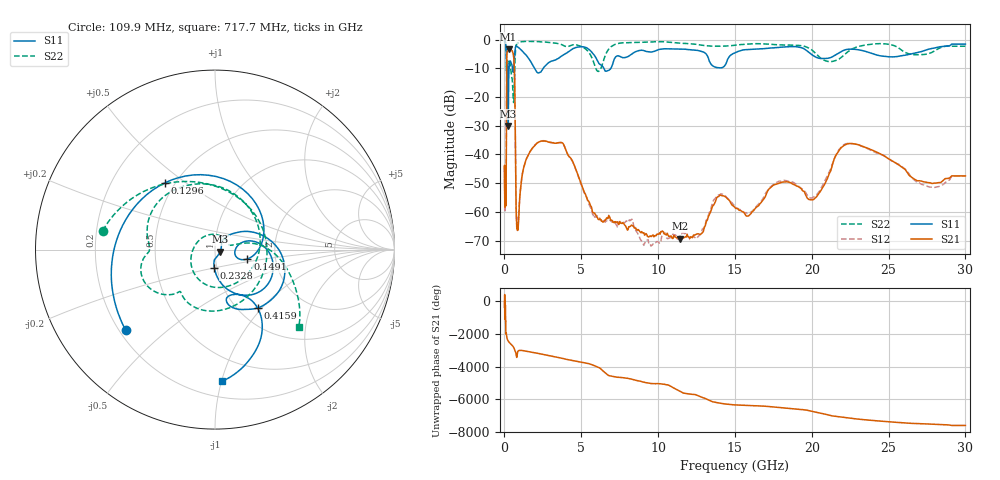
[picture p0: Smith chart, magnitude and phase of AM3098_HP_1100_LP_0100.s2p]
! Date/Time: Thu, Feb 28, 2019 8:44 AM
! Network Analyzer: Agilent Technologies E8364B Rev: A.07.50.67
! Sweep from 0.010 to 30.000 GHz, 1601 Points, Sweep Type: LOG
! Power Supply: 5.023 V, 0.002 A
# Hz S DB R 50
!freq MagS11 AngS11 MagS21 AngS21 MagS12 AngS12 MagS22 AngS22
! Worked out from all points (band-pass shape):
!   1601 points, 10 MHz to 30 GHz, reference 50 ohm
!   highest |S21| = -3.36 dB at 266.5 MHz (marker M1); lowest = -69.4 dB at 11.42 GHz (marker M2)
!   |S21| within 3 dB of the highest: 148.5 MHz to 606.2 MHz (457.7 MHz wide, 121 % of centre)
!   lowest |S11| = -30.1 dB at 246 MHz (marker M3), VSWR 1.06, Z = 53 - j1.29 ohm
!   |S11| at or under -10 dB: 205.2 MHz to 299.2 MHz (93.93 MHz wide, 37.2 % of centre); 1.96 GHz to 2.529 GHz (569.2 MHz wide, 25.4 % of centre); 6.464 GHz to 6.93 GHz (466 MHz wide, 6.96 % of centre)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
!   |S22| runs from -21.9 to -0.5 dB; largest |S21 - S12| = 0.011
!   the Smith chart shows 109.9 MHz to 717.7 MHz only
!   S11 on the Smith chart (normalised r, x): 109.9 MHz: 0.23, -0.37; 129.6 MHz: 0.44, +0.42; 149.1 MHz: 1.43, -0.15; 232.8 MHz: 0.97, -0.20; 415.9 MHz: 1.22, -0.95; 717.7 MHz: 0.32, -1.00
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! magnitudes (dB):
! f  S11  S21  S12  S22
! 10 MHz  -0.3  -44.2  -46.1  -0.5
! 38.04 MHz  -0.4  -57.3  -56.0  -0.7
! 109.9 MHz  -3.5  -51.5  -51.0  -4.0
! 129.6 MHz  -6.6  -21.4  -21.4  -10.6
! 144.7 MHz  -11.8  -7.5  -7.5  -9.4
! 149.1 MHz  -14.5  -6.2  -6.2  -10.0
! 232.8 MHz  -20.0  -3.4  -3.4  -8.6
! 246 MHz  -30.1  -3.4  -3.3  -8.7
! 266.5 MHz  -16.7  -3.4  -3.3  -8.6
! 415.9 MHz  -7.9  -3.6  -3.6  -10.7
! 550.5 MHz  -11.1  -4.6  -4.6  -18.7
! 649.3 MHz  -6.5  -10.9  -10.8  -14.7
! 717.7 MHz  -2.7  -40.4  -40.3  -3.9
! 773.6 MHz  -2.3  -61.6  -63.2  -1.9
! 863.6 MHz  -2.6  -66.3  -64.0  -1.1
! 2.084 GHz  -11.2  -36.3  -36.2  -0.7
! 3.779 GHz  -5.5  -36.0  -36.1  -1.9
! 7.926 GHz  -6.2  -65.4  -63.2  -1.1
! 11.42 GHz  -3.3  -69.4  -68.6  -1.3
! 20.2 GHz  -6.0  -55.3  -54.5  -4.6
! 22.56 GHz  -3.4  -36.2  -36.2  -3.5
! 30 GHz  -1.6  -47.5  -47.5  -2.3
